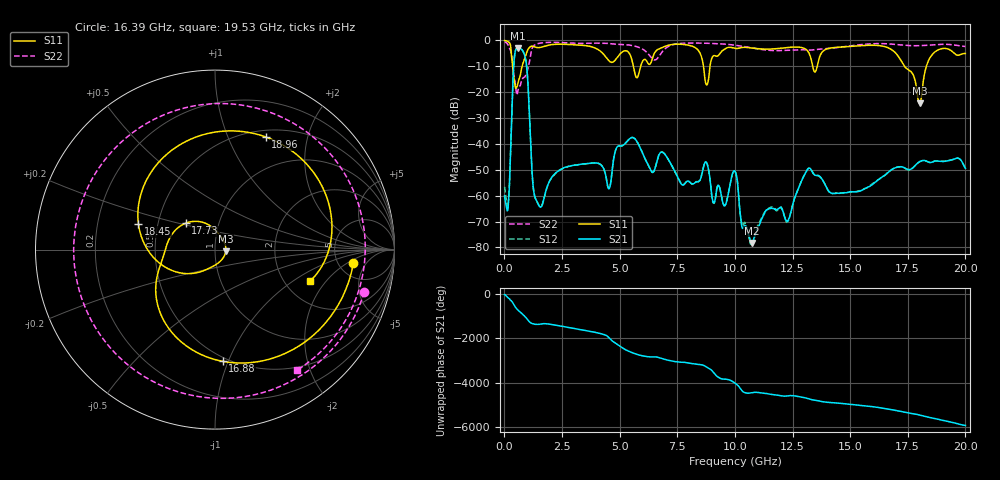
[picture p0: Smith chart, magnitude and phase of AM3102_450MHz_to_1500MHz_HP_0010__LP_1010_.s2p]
!Agilent Technologies,E8364B,MY43040894,A.07.50.67
!Agilent E8364B: A.07.50.67
!Date: Thursday, January 11, 2018 05:28:15
!Correction: S11(Full 2 Port(1,2))
!S21(Full 2 Port(1,2))
!S12(Full 2 Port(1,2))
!S22(Full 2 Port(1,2))
!S2P File: Measurements: S11, S21, S12, S22:
# Hz S  dB  R 50
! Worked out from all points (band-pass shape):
!   1601 points, 10 MHz to 20 GHz, reference 50 ohm
!   highest |S21| = -2.95 dB at 597.2 MHz (marker M1); lowest = -78.3 dB at 10.74 GHz (marker M2)
!   |S21| within 3 dB of the highest: 442.2 MHz to 884.4 MHz (442.2 MHz wide, 66.7 % of centre)
!   lowest |S11| = -24.4 dB at 18.01 GHz (marker M3), VSWR 1.13, Z = 56.3 - j1.05 ohm
!   |S11| at or under -10 dB: 356.2 MHz to 769.6 MHz (413.4 MHz wide, 73.4 % of centre); 5.595 GHz to 5.915 GHz (320 MHz wide, 5.56 % of centre); 17.36 GHz to 18.31 GHz (952.6 MHz wide, 5.34 % of centre)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
!   |S22| runs from -21.1 to -0.5 dB; largest |S21 - S12| = 0.0036
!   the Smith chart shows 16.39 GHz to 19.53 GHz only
!   S11 on the Smith chart (normalised r, x): 16.39 GHz: 6.93, -2.55; 16.88 GHz: 0.47, -0.95; 17.73 GHz: 0.69, +0.21; 18.45 GHz: 0.39, +0.14; 18.96 GHz: 0.58, +1.38; 19.53 GHz: 2.74, -1.39
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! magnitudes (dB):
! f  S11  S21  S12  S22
! 10 MHz  -0.1  -60.1  -56.6  -0.5
! 172.4 MHz  -0.6  -63.1  -62.6  -2.0
! 422.3 MHz  -15.1  -7.8  -7.8  -13.9
! 597.2 MHz  -16.1  -3.0  -3.0  -19.0
! 934.5 MHz  -5.5  -8.0  -7.9  -13.3
! 1.447 GHz  -2.8  -63.0  -62.9  -1.3
! 3.346 GHz  -1.9  -47.8  -47.8  -1.2
! 6.682 GHz  -3.4  -44.8  -44.7  -6.5
! 8.781 GHz  -17.2  -47.4  -47.3  -1.1
! 9.543 GHz  -3.5  -63.9  -63.8  -1.4
! 10.01 GHz  -3.1  -50.6  -50.6  -1.9
! 10.74 GHz  -3.0  -78.3  -79.3  -2.9
! 13.34 GHz  -8.6  -50.5  -50.5  -3.7
! 16.39 GHz  -2.2  -52.7  -52.9  -1.3
! 16.68 GHz  -3.0  -50.8  -50.7  -1.4
! 16.88 GHz  -4.1  -49.5  -49.5  -1.5
! 17.73 GHz  -13.2  -49.2  -49.2  -2.1
! 18.01 GHz  -24.4  -46.8  -46.9  -2.1
! 18.45 GHz  -6.9  -47.2  -47.2  -1.8
! 18.96 GHz  -3.2  -46.8  -46.7  -1.5
! 19.53 GHz  -5.1  -45.8  -45.8  -1.8
! 20 GHz  -5.1  -49.4  -49.3  -2.4
